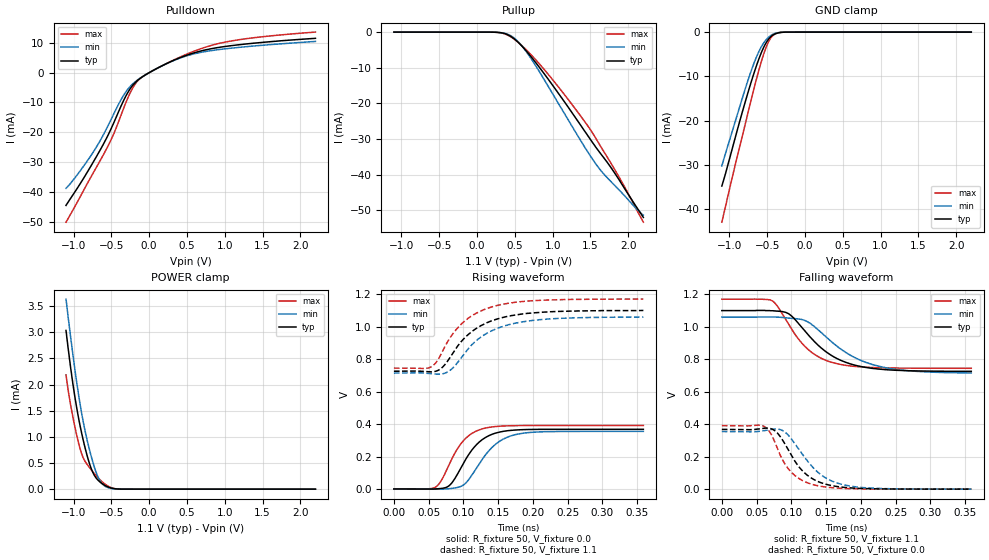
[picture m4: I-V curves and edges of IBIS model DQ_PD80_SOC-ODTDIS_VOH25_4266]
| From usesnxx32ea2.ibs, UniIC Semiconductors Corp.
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| DQ_PD80_SOC-ODTDIS_VOH25_4266
| (80 Ohm Pulldown, SOC ODT disabled setting, VOH=VDDQ/2.5 cal. point, 3200-4266Mbps)
[Model]   DQ_PD80_SOC-ODTDIS_VOH25_4266
Model_type   I/O
Vinl = 160.000mV
Vinh = 280.000mV
Vmeas = 220.000mV
Vref = 0.0mV
Cref = 0.0pF
|   typ   min   max
|C_comp   0.834pF   0.784pF   0.884pF
C_comp_pullup   0.4170pF   0.3920pF   0.4420pF
C_comp_pulldown   0.4170pF   0.3920pF   0.4420pF
| Note: C_comp changes when the ODT circuit is enabled.
[Model Spec]
| Input threshold voltage corners
Vinl   0.1600V   0.1520V   0.1740V
Vinh   0.2800V   0.2720V   0.2940V
| Measurement voltage corners
Vmeas   0.2200V   0.2120V   0.2340V
| Timing spec test load voltage corners
Vref   0.0000V   0.0000V   0.0000V
| Dynamic Overshoot Parameters from LPDDR4 Specification
D_overshoot_ampl_h   0.30   NA   NA
D_overshoot_ampl_l   0.30   NA   NA
D_overshoot_area_h   0.1n   NA   NA
D_overshoot_area_l   0.1n   NA   NA
[Voltage Range]   1.1000V   1.0600V   1.1700V
[Pullup Reference]   1.1000V   1.0600V   1.1700V
| Junction Temperature (Ambient temp is 35C typ 95C min -40C max)
[Temperature Range]   50.0   110.0   -40.0
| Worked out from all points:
|   slope of the pulldown table from 0 to 0.165 V, typ, clamps not added: 73.9 ohm
|   slope of the pullup table from 0 to 0.165 V, typ, clamps not added: 17.7 kohm
|   GND clamp passes 1 mA (typ) near -0.45 V on its own axis
|   POWER clamp passes 1 mA (typ) near -0.88 V on its own axis
|   rising waveform, R_fixture 50, V_fixture 0.0: 20-80 % time 35.1ps typ, 38.9ps min, 32ps max; typ from 0.001 V to 0.368 V
|   falling waveform, R_fixture 50, V_fixture 1.1: 20-80 % time 58ps typ, 69ps min, 47.3ps max; typ from 1.1 V to 0.726 V
|   rising waveform, R_fixture 50, V_fixture 1.1: 20-80 % time 54.9ps typ, 56.7ps min, 51.7ps max; typ from 0.726 V to 1.1 V
|   falling waveform, R_fixture 50, V_fixture 0.0: 20-80 % time 38.3ps typ, 44.3ps min, 32.9ps max; typ from 0.368 V to 0.001 V
[Pulldown]
|   Voltage   I(typ)   I(min)   I(max)
-1.1V     -44.48mA   -38.75mA   -50.09mA
-892.1mV  -36.4mA    -32.2mA    -40.64mA
-704mV    -28.42mA   -25.19mA   -31.99mA
-492.8mV  -18.21mA   -15.13mA   -21.9mA
-383.9mV  -11.9mA    -9.616mA   -15.05mA
-311.3mV  -8.018mA   -6.571mA   -10.27mA
-202.4mV  -3.82mA    -3.443mA   -4.514mA
-100.1mV  -1.592mA   -1.543mA   -1.618mA
391.6mV   4.819mA    4.708mA    5.003mA
847mV     8.116mA    7.448mA    9.269mA
1.292V    9.612mA    8.694mA    11.38mA
2.2V      11.48mA    10.44mA    13.57mA
[GND Clamp]
|   Voltage   I(typ)   I(min)   I(max)
-1.1V     -34.75mA   -30.2mA    -42.92mA
-1.05V    -31.86mA   -27.33mA   -39.27mA
-941.6mV  -25.02mA   -21.25mA   -31.32mA
-786.5mV  -15.53mA   -12.6mA    -20.5mA
-664.4mV  -8.74mA    -6.576mA   -12.08mA
-591.8mV  -5.258mA   -3.788mA   -7.5mA
-522.5mV  -2.666mA   -1.906mA   -3.813mA
-469.7mV  -1.357mA   -986.7uA   -1.787mA
-416.9mV  -598uA     -442.2uA   -665.2uA
-350.9mV  -166.4uA   -126.3uA   -147.4uA
-258.5mV  -16.15uA   -14.14uA   -9.927uA
2.2V      0A         0A         0A
[Pullup]
|   Voltage   I(typ)   I(min)   I(max)
-1.1V     4.106uA    7.431uA    1.361uA
266.2mV   -69.17uA   -67.98uA   -71.79uA
388.3mV   -576.1uA   -478.3uA   -687.4uA
497.2mV   -1.982mA   -1.772mA   -2.09mA
599.5mV   -4.068mA   -4.034mA   -3.93mA
734.8mV   -7.452mA   -8.085mA   -6.824mA
1.025V    -15.68mA   -18.21mA   -14.03mA
1.448V    -28.55mA   -33.09mA   -25.83mA
1.566V    -32.18mA   -36.88mA   -29.66mA
1.685V    -35.54mA   -40.05mA   -33.84mA
1.956V    -44.08mA   -46.07mA   -43.63mA
2.2V      -52.05mA   -51.39mA   -53.39mA
[POWER Clamp]
|   Voltage   I(typ)   I(min)   I(max)
-1.1V     3.033mA    3.633mA    2.184mA
-1.041V   2.345mA    2.929mA    1.625mA
-977.9mV  1.723mA    2.241mA    1.16mA
-911.9mV  1.2mA      1.611mA    764.4uA
-852.5mV  818.1uA    1.148mA    543.5uA
-776.6mV  434.1uA    683.3uA    390.2uA
-707.3mV  225.4uA    345.5uA    267.6uA
-651.2mV  138.6uA    162.3uA    181.2uA
-591.8mV  77.94uA    64.81uA    105.5uA
-496.1mV  20.04uA    12.32uA    25.73uA
-393.8mV  2.196uA    1.489uA    1.934uA
2.2V      0A         0A         0A
[Ramp]
|   typ   min   max
| 20% - 80%
dV/dt_r   220.51m/35.12p   212.86m/38.87p   234.61m/31.95p
dV/dt_f   224.46m/57.99p   206.41m/68.96p   255.16m/47.24p
| 25% - 75%
|dV/dt_r   183.76m/27.95p   177.38m/30.96p   195.51m/25.38p
|dV/dt_f   187.05m/46.15p   172.01m/54.89p   212.64m/37.50p
R_load = 50
[Rising Waveform]
R_fixture = 50
V_fixture = 0.0
|   Time   V(typ)   V(min)   V(max)
0s        836.2uV    685.8uV    613uV
58ps      506.9uV    -45.3uV    7.832mV
67ps      3.418mV    -439.2uV   44.62mV
77ps      13.93mV    1.482mV    127.9mV
86ps      53.46mV    5.803mV    207.8mV
102ps     173.7mV    31.95mV    306.9mV
129ps     310.1mV    194.6mV    373mV
152ps     351mV      294.2mV    387.2mV
181ps     365.2mV    340.8mV    391mV
359ps     368.4mV    355.4mV    391.6mV
[Falling Waveform]
R_fixture   = 50
V_fixture   = 1.1
V_fixture_min = 1.06
V_fixture_max = 1.17
|   Time   V(typ)   V(min)   V(max)
0s        1.1V       1.06V      1.17V
73ps      1.099V     1.061V     1.159V
96ps      1.081V     1.054V     1.016V
118ps     982.4mV    1.041V     886.3mV
137ps     893.3mV    987.8mV    820.4mV
157ps     825.9mV    911.1mV    782.9mV
191ps     764.5mV    811.4mV    756.4mV
230ps     738.2mV    753.4mV    747.8mV
284ps     728.3mV    724.8mV    745.2mV
359ps     725.9mV    716mV      744.7mV
[Rising Waveform]
R_fixture   = 50
V_fixture   = 1.1
V_fixture_min = 1.06
V_fixture_max = 1.17
|   Time   V(typ)   V(min)   V(max)
0s        725.5mV    714.2mV    744.7mV
53ps      721.5mV    710.7mV    751.4mV
62ps      728.2mV    707.5mV    787.3mV
75ps      774.9mV    716.2mV    890.4mV
89ps      864.6mV    765.3mV    979mV
107ps     951.9mV    864.6mV    1.052V
124ps     1.003V     932.4mV    1.095V
145ps     1.042V     982.9mV    1.127V
209ps     1.088V     1.043V     1.162V
359ps     1.1V       1.059V     1.17V
[Falling Waveform]
R_fixture = 50
V_fixture = 0.0
|   Time   V(typ)   V(min)   V(max)
0s        368.5mV    355.6mV    391.7mV
58ps      374.4mV    359mV      391.8mV
74ps      367mV      370.3mV    313.1mV
86ps      312.3mV    364.2mV    192.4mV
98ps      224.6mV    321.2mV    114.5mV
114ps     122.9mV    226.6mV    58.43mV
132ps     61.05mV    130.3mV    27.72mV
157ps     23.47mV    52.97mV    10.16mV
191ps     6.912mV    15.81mV    2.96mV
359ps     897.5uV    805.7uV    637uV
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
